(* SV publisher APDU *)
{attribute 'call_after_init'}
{attribute 'analysis' := '-33'}
{attribute 'no_assign'}
{attribute 'no_explicit_call' := 'Direct call not allowed for type FB_SVTXAPDU_IED_MUnn_LLN0_MSVCB02'}
FUNCTION_BLOCK FB_SVTXAPDU_IED_MUnn_LLN0_MSVCB02 EXTENDS FB_GseSvApduClass
VAR_INPUT
	TxData: ST_SVAPDU_IED_MUnn_LLN0_MSVCB02; (* SV data to be published in TwinCAT PLC host format (little endian) *)
END_VAR
VAR
	Asdu1: ARRAY [0..cOversampleFactor_IED_MUnn_LLN0_MSVCB02_Asdu1-1] OF FB_SVTXASDU_IED_MUnn_LLN0_MSVCB02;
	index: UINT(0..cOversampleFactor_IED_MUnn_LLN0_MSVCB02_Asdu1-1);
END_VAR

{attribute 'call_after_init'}
(* This method adds new oversampling ASDU to the APDU *)
METHOD FINAL AddArrayOfAsduToContainer
VAR
END_VAR
FOR index:=0 TO cOversampleFactor_IED_MUnn_LLN0_MSVCB02_Asdu1-1 BY 1 DO
	Asdu1[index].index:=index;
	Asdu1[index].ipApdu:=THIS^.AddAsduToContainer(ipAsdu:=Asdu1[index]);
END_FOR
END_METHOD

{attribute 'analysis' := '-33'}
(* Converts SV publisher data to be sent from host (little-endian) to network (big-endian) byte order *)
METHOD FINAL OnSvPublisherHostToNet
VAR_INPUT
	ipAdapter: I_GseAdapterClass; (* Network adapter interface pointer *)
	ipApdu: I_GseSvApduClass; (* APDU object interface pointer *)
END_VAR
VAR
END_VAR
FOR index:=0 TO cOversampleFactor_IED_MUnn_LLN0_MSVCB02_Asdu1-1 BY 1 DO
	Asdu1[index].nSmpCnt:= TxData.Asdu1.nSmpCnt[index]; (* Set sample counter *)
	Asdu1[index].eSmpSynch:= TxData.Asdu1.eSmpSynch[index]; (* Set synchronization type: 0..2 *)
	Asdu1[index].tRefrTm:= TxData.Asdu1.tRefrTm[index]; (* Set refresh time stamp (optional) *)

	(* Convert SV data to be sent from host byte order to network byte order *)
	HostToNetInt32(in:=TxData.Asdu1.IED_MUnn_InnATCTR1_AmpSv_instMag_i[index], out:=Asdu1[index].Values.IED_MUnn_InnATCTR1_AmpSv_instMag_i);
	HostToNetQuality(in:=TxData.Asdu1.IED_MUnn_InnATCTR1_AmpSv_q[index], out:=Asdu1[index].Values.IED_MUnn_InnATCTR1_AmpSv_q);
	HostToNetInt32(in:=TxData.Asdu1.IED_MUnn_InnBTCTR2_AmpSv_instMag_i[index], out:=Asdu1[index].Values.IED_MUnn_InnBTCTR2_AmpSv_instMag_i);
	HostToNetQuality(in:=TxData.Asdu1.IED_MUnn_InnBTCTR2_AmpSv_q[index], out:=Asdu1[index].Values.IED_MUnn_InnBTCTR2_AmpSv_q);
	HostToNetInt32(in:=TxData.Asdu1.IED_MUnn_InnCTCTR3_AmpSv_instMag_i[index], out:=Asdu1[index].Values.IED_MUnn_InnCTCTR3_AmpSv_instMag_i);
	HostToNetQuality(in:=TxData.Asdu1.IED_MUnn_InnCTCTR3_AmpSv_q[index], out:=Asdu1[index].Values.IED_MUnn_InnCTCTR3_AmpSv_q);
	HostToNetInt32(in:=TxData.Asdu1.IED_MUnn_InnNTCTR4_AmpSv_instMag_i[index], out:=Asdu1[index].Values.IED_MUnn_InnNTCTR4_AmpSv_instMag_i);
	HostToNetQuality(in:=TxData.Asdu1.IED_MUnn_InnNTCTR4_AmpSv_q[index], out:=Asdu1[index].Values.IED_MUnn_InnNTCTR4_AmpSv_q);
	HostToNetInt32(in:=TxData.Asdu1.IED_MUnn_UnnATVTR1_VolSv_instMag_i[index], out:=Asdu1[index].Values.IED_MUnn_UnnATVTR1_VolSv_instMag_i);
	HostToNetQuality(in:=TxData.Asdu1.IED_MUnn_UnnATVTR1_VolSv_q[index], out:=Asdu1[index].Values.IED_MUnn_UnnATVTR1_VolSv_q);
	HostToNetInt32(in:=TxData.Asdu1.IED_MUnn_UnnBTVTR2_VolSv_instMag_i[index], out:=Asdu1[index].Values.IED_MUnn_UnnBTVTR2_VolSv_instMag_i);
	HostToNetQuality(in:=TxData.Asdu1.IED_MUnn_UnnBTVTR2_VolSv_q[index], out:=Asdu1[index].Values.IED_MUnn_UnnBTVTR2_VolSv_q);
	HostToNetInt32(in:=TxData.Asdu1.IED_MUnn_UnnCTVTR3_VolSv_instMag_i[index], out:=Asdu1[index].Values.IED_MUnn_UnnCTVTR3_VolSv_instMag_i);
	HostToNetQuality(in:=TxData.Asdu1.IED_MUnn_UnnCTVTR3_VolSv_q[index], out:=Asdu1[index].Values.IED_MUnn_UnnCTVTR3_VolSv_q);
	HostToNetInt32(in:=TxData.Asdu1.IED_MUnn_UnnNTVTR4_VolSv_instMag_i[index], out:=Asdu1[index].Values.IED_MUnn_UnnNTVTR4_VolSv_instMag_i);
	HostToNetQuality(in:=TxData.Asdu1.IED_MUnn_UnnNTVTR4_VolSv_q[index], out:=Asdu1[index].Values.IED_MUnn_UnnNTVTR4_VolSv_q);
END_FOR
END_METHOD

END_FUNCTION_BLOCK
